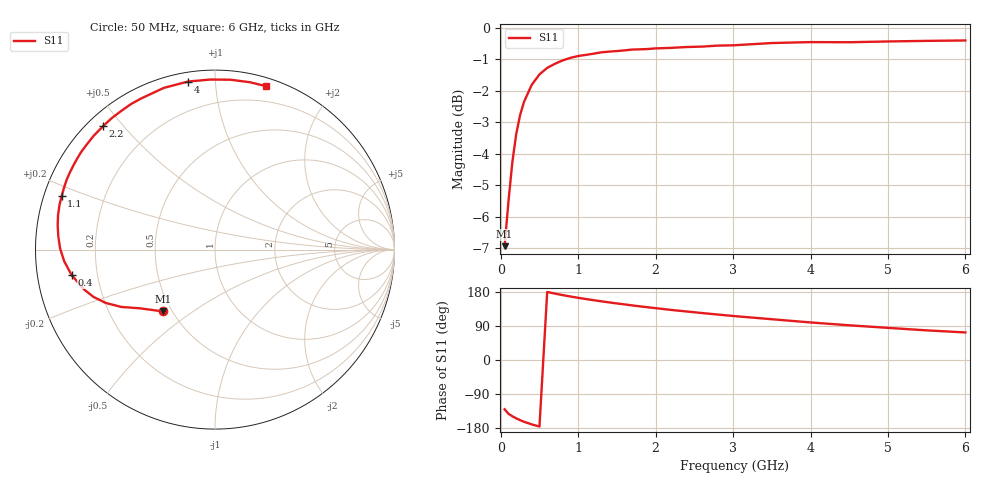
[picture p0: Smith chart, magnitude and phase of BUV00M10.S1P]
! Infineon Technologies  Discrete & RF Semiconductors
! BB 833
! Si Tuning Diode in SOD323
! VR =
! S-Parameters:  June  1999
# GHz  S  MA  R  50
!  f  S11
! GHz  MAG  ANG
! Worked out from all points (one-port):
!   34 points, 50 MHz to 6 GHz, reference 50 ohm
!   lowest |S11| = -6.9 dB at 50 MHz (marker M1), VSWR 2.64, Z = 22.4 - j19.4 ohm
!   |S11| at or under -10 dB: nowhere
!   S11 on the Smith chart (normalised r, x): 50 MHz: 0.45, -0.39; 400 MHz: 0.11, -0.09; 1.1 GHz: 0.05, +0.17; 2.2 GHz: 0.04, +0.44; 4 GHz: 0.05, +0.85; 6 GHz: 0.07, +1.36
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0.05  0.4498 -130.0
0.1  0.5302 -141.9
0.15  0.6116 -148.5
0.2  0.6777 -154.0
0.25  0.7263 -158.7
0.3  0.762 -163.0
0.4  0.8112 -169.9
0.5  0.8428 -175.6
0.6  0.863 179.6
0.7  0.8761 175.2
0.8  0.887 171.2
0.9  0.8953 167.6
1.1  0.905 160.8
1.3  0.9135 154.8
1.5  0.9177 149.2
1.6  0.92 146.7
1.7  0.9228 144.0
1.9  0.9246 139.1
2.2  0.9285 132.2
2.4  0.9314 128.0
2.8  0.9362 120.0
3  0.9372 116.2
3.5  0.945 107.6
4  0.9483 99.1
4.5  0.9478 91.6
5  0.9505 84.8
5.5  0.9525 78.2
6  0.954 72.7
